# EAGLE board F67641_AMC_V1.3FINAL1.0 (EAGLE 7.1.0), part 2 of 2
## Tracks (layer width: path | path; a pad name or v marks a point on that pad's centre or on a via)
+5..12V
  Top 0.406: C55.1 133.85,154.74 U3.3 | U3.1 135.28,152.84 135.74,153.3 135.74,154.64 C55.1 | C54.1 137.64,157.46 arc45 137.56,157.28 D6.1 D7.1 135.79,154.67 arc-45 C55.1
ACT  (via drill 0.4)
  Top 0.254: 117.74,138.48 112.19,144.18 | 112.19,144.18 107.6,148.88 107.6,166.33 100.71,173.22 100.71,173.27 59,173.27 LED_ACT.K 54.01,171.54 53.5,172.05 53.5,174.21 54.38,175.1 v58.3,175.1 | 112.19,144.18 117.86,138.51 117.86,104.64 109.86,96.64 U4.51
  Top 0.61: U5.2 39.27,177.2 42.82,180.75 65.4,180.8 ACT.2
  Bottom 0.254: v58.3,175.1 61.57,178.37 62.97,178.37 ACT.2
AGND_I1  (via drill 0.4)
  Top 0.813: U$13.2 140.64,29.69 C35.2 | U$16.7 140.57,44.4 C39.2 138.57,44.36 U$16.6 140.48,50.23 140.75,50.5
  other vias: 121.67,20.51 124.21,20.51 126.75,20.51 130.56,20.56 135.64,21.83 135.64,19.8 140.47,21.83 140.47,20.05 133.86,28.69 133.86,26.91 143.51,28.69 143.51,26.66 122.69,22.59 122.43,27.42 121.67,31.99 123.45,31.99 117.61,33.52 117.61,36.82 117.61,41.14 117.61,44.69 117.61,47.99 117.61,50.28 119.38,47.99 119.38,45.45 123.45,38.09 122.18,38.09 122.18,36.82 123.45,36.82 120.65,41.9 122.43,41.9 124.46,41.9 126.75,34.28 128.81,34.28 134.62,40.37 134.37,30.98 141.48,31.48 143.51,31.48 143.51,33.52 143.51,37.83 140.97,37.83 140.97,39.87 143.51,39.87 129.62,51.42 130.84,51.42 132.06,51.42 133.28,51.42 129.62,50.46 130.84,50.46 132.06,50.46 133.28,50.46 129.87,43.04 134.5,50.31 128.78,38.09 130.18,38.14 131.55,38.11 133.68,38.06 128.81,35.73 130.23,35.73 131.5,35.73 133.71,35.73
  pour Bottom: 115.9,52.16 144.53,52.16 144.53,17.89 115.9,17.89
  pour Top: 115.9,52.16 144.53,52.16 144.53,17.89 115.9,17.89
AGND_I2  (via drill 0.4)
  Top 0.813: U$7.2 90.64,29.69 C44.2 | U$8.7 90.57,44.4 C45.2 88.57,44.36 U$8.6 90.73,50.23 90.76,50.25
  other vias: 70.87,20.51 74.43,20.51 72.65,22.59 76.97,20.51 81.03,20.51 84.33,31.23 91.19,31.48 93.48,31.48 93.48,34.02 93.48,37.07 91.19,37.07 91.19,39.87 93.48,39.87 83.87,40.12 84.84,49.26 72.39,28.44 71.89,31.99 73.41,31.99 72.14,36.82 73.16,36.82 72.14,39.1 73.16,39.1 70.87,41.9 72.65,41.9 74.43,41.9 76.71,34.53 79.25,34.53 67.06,37.33 67.06,41.39 67.06,44.18 69.35,45.45 69.35,47.74 67.06,47.74 67.06,49.77 85.09,20.31 90.68,20.05 85.09,22.09 90.68,22.09 84.2,26.4 84.18,28.69 93.48,26.15 93.48,28.69 79.53,51.42 80.75,51.42 81.97,51.42 83.19,51.42 79.53,50.46 80.75,50.46 81.97,50.46 83.19,50.46 79.96,43.09 79.2,37.81 80.6,37.81 81.72,37.78 79.23,35.93 80.6,35.9 81.74,35.9 83.87,38.04 83.93,35.7
  pour Bottom: 65.9,52.16 94.53,52.16 94.53,17.89 65.9,17.89
  pour Top: 65.9,52.16 94.53,52.16 94.53,17.89 65.9,17.89
AGND_I3  (via drill 0.4)
  Top 0.813: U$15.6 38.48,50.15 38.48,44.45 C50.2 40.57,44.4 U$15.7 | 40.82,50.18 40.7,50.3 | U$14.2 40.64,30.93 40.06,31.51 C48.2
  other vias: 22.81,42.05 24.67,42.05 20.6,42.05 21.85,39.79 21.87,36.95 42.73,39.18 42.65,36.01 40.49,36.01 40.54,39.18 17.4,44.56 17.4,47.28 17.4,49.52 17.4,33.16 27.49,33.64 28.96,39.1 17.4,36.67 17.4,41.24 30.79,39.1 29.77,33.64 34.93,49.31 30.51,20.51 26.88,20.51 23.91,20.51 21.01,20.51 18.83,20.51 19.79,47.41 19.79,45.15 30.33,42.69 33.74,31.1 34.22,41.44 24.29,49.31 23.37,39.79 23.37,36.95 21.87,32.12 23.42,32.14 22.66,29.1 22.64,22.49 42.65,33.19 40.62,33.19 42.65,31.84 34.9,22.19 40.75,22.19 40.75,19.9 34.9,19.9 42.65,27.27 42.65,28.99 33.74,26.51 33.74,29.05 29.42,51.42 30.64,51.4 29.42,50.46 30.64,50.46 31.86,51.4 31.86,50.46 33.07,51.4 33.07,50.46 28.91,35.5 30.1,35.5 31.17,35.52 28.91,37.88 30.15,37.86 31.2,37.86 33.1,37.86 33.1,35.85
  pour Bottom: 15.9,52.16 44.53,52.16 44.53,17.89 15.9,17.89
  pour Top: 15.9,52.16 44.53,52.16 44.53,17.89 15.9,17.89
AMC_CLKIN  (via drill 0.4)
  Top 0.254: 123.36,67.64 123.37,67.65 | U4.47 99.15,92.43 96.83,90.11 96.83,89.55
  Top 0.61: U$3.CLKIN 73.41,61.06 73.41,65.19 74.3,66.08 74.3,68.14 JP2.2 68.06,68.19 R16.2 | JP3.2 23.37,67.17 U$4.CLKIN | JP1.2 123.37,67.65 U$2.CLKIN | v94.87,77.9 96.83,79.86 96.83,89.55
  Bottom 1.016: 75.85,77.9 v94.87,77.9 122.05,77.9 124.67,75.28 JP1.2 | JP3.2 25,75.15 27.77,77.9 72.46,77.9 73.55,76.81 | JP2.2 74.25,76.11 | 74.25,76.11 74.25,76.3 75.85,77.9 | 73.55,76.81 74.25,76.11 | 69.52,77.9 74.64,77.9 | 75.85,77.9 74.64,77.9 | 74.64,77.9 73.55,76.81
AUXVCC1
  Top 0.254: C4.1 79.44,101.31 C5.1 82.99,101.31 R6.2 83.05,101.26 84.15,101.26 85.77,99.64 U4.19
AUXVCC2
  Top 0.254: 74.72,101.11 C7.1 | 74.74,101.13 C7.1 | C7.1 C6.1 77.86,101.34 R5.2 | U4.18 85.95,100.15 83.95,102.15 78.08,102.15 77.91,101.97 R5.2 | 77.91,101.35 R5.2
AUXVCC3
  Top 0.254: 91.28,92.22 C58.1 | 91.33,90.44 C59.1 | U4.26 88.66,93.83 89.13,93.36 90.14,93.36 C58.1 | C59.1 C58.1 | R7.2 91.25,90.33 C59.1
AVCC  (via drill 0.2, 0.6)
  Top 0.254: U4.9 83.84,104.64 81.79,106.69 C29.1
  Top 0.406: v44.67,108.35 D46.C | v44.67,98.85 D48.C | v44.67,117.85 D44.C
  Top 0.61: v44.67,108.35 R123.1 | v44.67,117.85 R117.1 | v44.67,98.85 R127.1
  Top 0.813: 44.67,97.35 v44.67,98.85 | C29.1 C31.1 75.12,108.33 56.3,127.16 R36.2 44.67,127.15 v44.67,125.85
  Bottom 0.813: v44.67,98.85 v44.67,108.35 v44.67,117.85 v44.67,125.85
AVDD_I1
  Top 0.61: D3.C 117.25,27.56 117.25,20.28 118.67,18.86 131.73,18.86 132.52,19.67 132.52,27.17 | U$2.AVDD 127.18,49.82 127.75,49.25 129.19,49.25 C12.1 CSEL1.1 130.97,47.28 132.52,45.75 132.52,28.16 | D4.C 131.9,27.64 131.91,27.65 132.01,27.65 | 132.01,27.65 132.52,28.16 | 132.52,27.17 132.01,27.65 | 132.52,28.16 132.52,27.17
AVDD_I2
  Top 0.61: 82.66,28.13 82.66,45.63 81,47.28 CSEL2.1 C19.1 79.25,49.19 77.96,49.19 77.18,49.96 U$3.AVDD | D1.C 67.06,27.37 67.06,20.16 68.25,18.96 81.84,18.96 82.66,19.77 82.66,26.99 82.13,27.51 82.13,27.61 | D5.C 78.08,27.61 82.13,27.61 | 82.13,27.61 82.66,28.13 | 82.66,27.09 82.66,28.13
AVDD_I3
  Top 0.61: D13.C 17.28,19.7 18.09,18.89 31.17,18.89 31.74,19.46 32.08,19.8 32.19,19.9 32.19,27.15 31.7,27.64 | U$4.AVDD 27.18,49.77 27.77,49.19 29.25,49.19 C21.1 CSEL3.1 30.79,47.28 32.19,45.89 32.19,28.13 | D15.C 31.7,27.64 | 31.7,27.64 32.19,28.13 | 32.19,28.13 32.19,27.06
BTN1
  Top 0.254: U4.46 98.64,95.96 98.86,96.18 103.41,96.18 105.72,93.86 R49.2
  Top 0.61: BTN1.2 122.1,93.85 118.93,93.85 R49.2
COM0  (via drill 0.2)
  Top 0.254: U4.32 91.66,96.91 94.75,100 94.75,107.25 v95.5,108
  Bottom 0.254: LCD1.COM0 94.49,161.57 106.25,161.57 112.75,155.07 112.75,111.5 108.5,107.25 98.5,107.25 97.5,108.25 95.75,108.25 v95.5,108
COM1  (via drill 0.2)
  Top 0.254: U4.33 92.17,96.67 95.25,99.75 95.25,106.5 96.25,107.5 v97.25,107.5
  Bottom 0.254: LCD1.COM1 96.53,162.07 106.5,162.07 113.25,155.32 113.25,111.25 108.75,106.75 98,106.75 v97.25,107.5
COM2  (via drill 0.2)
  Top 0.254: U4.34 92.65,96.4 96,99.75 96,106 v96.25,106.25
  Bottom 0.254: LCD1.COM2 98.57,162.57 106.75,162.57 113.75,155.57 113.75,111 109,106.25 v96.25,106.25
COM3  (via drill 0.2)
  Top 0.254: v97.25,105 96.75,105 96.5,104.75 96.5,99.5 93.16,96.16 U4.35
  Bottom 0.254: LCD1.COM3 100.61,163.07 105.25,163.07 106.98,163.09 114.25,155.82 114.25,110.75 109.2,105.7 97.97,105.7 97.27,105 v97.25,105
CUR1+
  Top 0.61: I1+.TP 120.68,23.23 D3.A D11.C 120.68,33.75 TVS2.C R/L9.2
CUR1+1
  Top 0.61: I2+.TP 70.68,23.23 D1.A D2.C 70.68,33.75 TVS1.C R/L1.2
CUR1+2
  Top 0.61: R/L3.2 TVS3.C 20.68,33.75 D14.C D13.A 20.68,23.23 I3+.TP
CUR1-
  Top 0.61: I1-.TP 124.65,23.14 D4.A 124.65,29.81 D12.C 124.62,33.87 TVS2.A R/L10.2
CUR1-1
  Top 0.61: I2-.TP 74.65,23.14 D5.A 74.62,27.67 D10.C 74.64,29.86 TVS1.A R/L2.2
CUR1-2
  Top 0.61: I3-.TP 24.65,23.14 D15.A 24.62,27.67 D35.C 24.62,33.87 TVS3.A R/L4.2
DRESET  (via drill 0.2)
  Top 0.254: U4.100 88.66,104.55 v91.88,101.33
  Bottom 0.254: v91.88,101.33 94.64,98.56 126.16,98.56 arc-45 126.34,98.49 128.43,96.41 128.43,89.65 131.07,87.01 131.5,87.01 137.42,87.01 JP5.2
DTCK  (via drill 0.2)
  Top 0.254: U4.99 89.14,105.06 v91.37,102.83
  Bottom 0.254: JP6.2 137.44,89.67 129.7,89.67 129.11,90.26 129.11,97.07 127.05,99.13 arc45 126.87,99.2 95.03,99.2 94.85,99.38 94.85,99.4 91.42,102.83 v91.37,102.83
DTDI  (via drill 0.2)
  Top 0.254: U4.97 90.16,106.48 v93.22,103.42
  Bottom 0.254: JP8.2 137.39,94.96 133.63,94.96 132.03,94.96 130.84,96.15 130.84,98.95 129.52,100.27 arc45 129.34,100.34 96.3,100.34 v93.22,103.42
DTDO  (via drill 0.2)
  Top 0.254: U4.96 90.67,107.22 v93.3,104.53
  Bottom 0.254: JP9.2 137.47,97.68 133.21,97.68 arc-45 133.03,97.75 126.47,104.31 115.58,104.31 arc45 115.4,104.23 112.12,100.95 96.85,100.95 95.46,102.35 95.46,102.38 v93.3,104.53
DTMS  (via drill 0.2)
  Top 0.254: U4.98 89.65,105.92 v91.5,104.08
  Bottom 0.254: JP7.2 137.6,92.5 133.35,92.5 130.71,92.5 129.95,93.26 129.95,97.85 128.15,99.66 arc45 127.97,99.73 95.79,99.73 95.18,100.34 95.18,100.37 91.5,104.05 v91.5,104.08
DVCC  (via drill 0.2, 0.4, 0.6)
  Top 0.254: U4.21 84.82,98.65 84.43,98.26 84.43,95.72 82.83,94.12 78.29,94.12 77.96,94.45 C17.1
  Top 0.406: v60.27,166.27 R58.1 | v70.27,166.27 R22.1 | v80.27,166.27 R57.1 | v90.27,166.27 R21.1 | v100.27,166.27 R20.1 | 90.53,61.07 U$8.2 | U$2.DVDD 122.1,61.9 | 122,63.48 C24.1 | 140.57,63.17 C51.1 140.5,63.24 | 80.32,177.23 80.35,177.26 80.81,177.26 arc-45 80.88,177.23 | 128.86,109.4 arc-45 128.79,109.43 128.39,109.83 | 128.86,109.53 128.86,110.32 arc45 128.78,110.5 | 128.25,109.97 128.25,110.3 arc-45 128.32,110.48 128.86,111.01 | 121.64,128.08 v121.62,128.11 121.71,128.02 C65.2 138.38,128.09 U1.1
  Top 0.61: 90.53,61.07 C46.1 90.53,64.61 90.03,65.1 U$6.2 90.03,66.98 89.72,67.3 84.63,67.3 C47.1 84.43,67.19 84.43,69.51 v84.46,69.53 | U$8.2 U$8.3 | 71.86,63.23 C26.1 | v120.73,68.31 122.09,66.96 C23.1 C24.1 122.1,63.55 122.1,61.9 | v107.06,80.58 v107.06,73.88 107.19,74 132.34,74 134.48,71.86 C42.1 139.68,67.2 139.75,67.27 140.03,66.99 U$10.2 140.03,65.29 140.49,64.83 140.49,63.24 C51.1 | 71.83,66.74 v71.91,66.81 | 68.51,80.28 68.79,80.56 | 71.85,66.75 v71.91,66.81 | C22.1 59.41,66.86 CLOCK_GENERATOR.4 59.43,68.53 v59.34,68.62 | U$15.3 U$15.2 40.57,63.17 C41.1 | 40.5,63.24 C41.1 | U$16.3 U$16.2 140.5,61.1 140.5,63.24 | C41.1 40.52,63.22 40.52,64.53 40.03,65.01 U$12.2 40.03,67.02 39.68,67.37 36.63,67.37 35.11,65.85 33.82,65.85 C52.1 33.73,65.94 v33.73,68.01 | U$4.DVDD C34.1 C27.1 22.11,70.51 23.93,72.33 33.71,72.33 v33.79,72.4 33.79,77.69 | 60.63,80.56 59.36,79.29 59.36,79.39 58.17,80.58 | v71.91,74.51 71.91,78.98 | 71.91,78.98 71.99,79.06 72.14,79.06 | 71.91,78.98 71.86,78.98 70.23,80.56 | 72.14,79.06 73.64,80.58 | 72.14,79.36 71.4,80.1 71.35,80.1 | 72.14,79.36 72.14,79.8 72.9,80.56 | 72.14,79.06 72.14,79.36 | v59.39,74.72 59.39,80.45 60,80.56 60.23,80.56 | v84.46,76.29 84.46,80.56 v84.43,80.58 | v71.91,66.81 72.04,66.69 C25.1 72.06,64.94 C26.1 | U$3.DVDD 72.1,63.22 C26.1 | U5.1 38.7,175.93 C66.1 40.56,176 41.53,175.02 41.53,173.34 42.27,172.61 43.82,172.61 43.84,172.63 | 44.66,171.87 44.66,173.16 44.52,173.31
  Top 0.813: DVCC.1 DVCC.2 DVCC.3 DVCC.4
  Top 1.27: 78.57,177.23 52.35,177.26 48.01,177.26 44.66,174.47 44.66,173.45 44.52,173.31 43.84,172.63 44.66,171.82 v44.66,166.05 R36.1 | 78.57,177.23 80.32,177.23 | 61.93,82.69 61.93,90.49 66.65,95.21 C16.1 C17.1 | 61.93,82.69 61.93,82.51 60.23,80.56 60.63,80.56 62.82,80.56 | 33.79,77.69 36.66,80.56 60,80.56 | 70.23,80.56 68.79,80.56 66.6,80.56 | v84.43,80.58 73.64,80.58 73.56,80.56 | 73.46,80.56 72.9,80.56 69.68,80.56 | DVCC.1 80.35,179.06 | 80.35,179.06 82.17,177.23 | 80.35,179.06 80.35,179.01 78.57,177.23 | 79.81,178.04 80.55,178.04 80.57,178.02 80.37,177.81 80.37,177.23 80.88,177.23 82.17,177.23 | R51.1 arc45 131.5,95.84 131.5,98.56 128.93,101.13 arc-45 128.86,101.31 128.86,109.4 | 127.62,110.6 127.5,110.48 arc-45 127.32,110.4 121.52,110.4 118.91,107.8 v118.91,97 R49.1 118.85,95.5 | 127.62,110.6 128.86,111.86 128.86,113.55 130.61,115.28 JP10.2 arc45 133.69,115.25 135.39,115.25 | 128.7,109.52 128.39,109.83 128.25,109.97 127.62,110.6 | 128.86,112.18 128.86,111.01 128.86,109.53 arc-45 128.66,109.61 | 82.17,177.23 102.39,177.28 109.53,177.28 v117.3,169.51 | 44.66,173.72 44.66,171.87 | 61.93,82.69 66.6,80.56 | 66.6,80.56 62.82,80.56 | 62.82,80.56 61.67,81.7
  Bottom 0.406: v121.62,128.11 118.01,128.11 117.2,128.92
  Bottom 0.61: v33.73,68.01 33.73,72.35 v33.79,72.4 | v71.91,66.81 v71.91,74.51 | v84.46,69.53 v84.46,76.29 | v59.34,68.62 59.34,74.66 v59.39,74.72 | v107.06,73.88 107.06,70.4 109.15,68.31 v120.73,68.31 | v44.66,166.05 44.88,166.27 v60.27,166.27 v70.27,166.27 v80.27,166.27 v90.27,166.27 v100.27,166.27
  Bottom 1.27: v84.43,80.58 v107.06,80.58 111.75,80.58 113.75,82.58 113.75,95.25 115.5,97 v118.91,97 | JP10.2 119.79,115.28 117.2,117.87 117.2,126.89 | 117.2,126.89 118.32,128 | v117.3,169.51 117.3,129.49 | 117.3,129.49 118.32,128 | 117.3,129.49 117.2,128.92 117.2,126.89 | 118.32,128 117.83,128 117.4,128.44
EXT
  Top 1.27: JTAG.4 152.23,101.87 153.44,103.09 153.44,107.25 148.95,111.75 142.14,111.75 136.15,117.74 arc45 135.97,117.82 JP10.3
EXT1
  Top 0.813: U$13.1 135.56,30.15 C35.1 136.93,35.06 AMC1PWR.1
EXT2
  Top 0.813: U$7.1 85.56,30.15 C44.1 86.92,35.06 AMC2PWR.1
EXT3
  Top 0.305: 37.04,31.62 C48.1
  Top 0.813: U$14.1 35.56,30.15 C48.1 | 37.04,31.62 AMC3PWR.1
GND  (via drill 0.3, 0.4)
  Top 0.254: 86.39,105.12 U4.8 84.5,105.12 83.77,105.86 83.77,106.9 v83.52,107.15 | U4.22 88.52,98.14 v88.87,97.79 | C65.1 138.36,124.04 138.33,124.02
  Top 0.406: U1.4 142.19,124.4
  Top 1.016: L6.2 30.6,82.1 37.25,88.75
  other vias: 71.75,150.07 59.25,150.07 84.25,143.07 71.75,143.07 59.25,143.07 80.76,120.63 50.34,91.5 38.51,82.23 38.51,84.23 38.51,86.72 40.46,82.23 40.46,84.23 40.46,86.72 42.26,82.23 42.26,84.23 42.26,86.72 103.96,183.59 76.93,182.67 42.09,126.12 42.09,124.87 42.1,123.8 41.92,110.28 24.52,63 20.27,66.75 20.27,68 27.02,63 27.02,65 29.02,63 29.02,65 29.64,61.27 31.52,61.25 42.77,65.43 33.02,62.25 46.01,65.43 37.77,66.25 36.14,69 42.77,68.5 37.02,63.25 66.49,63.09 66.49,65.2 78.52,63 78.27,64.5 79.52,61.75 79.77,63.75 86.52,63.25 75.02,64 80.77,61 82.02,61 86.52,69.75 86.77,66 95.66,69.67 95.66,66.75 116.49,66.75 116.49,63.29 124.77,64.25 128.27,65 129.77,65 128.27,63.75 129.77,63.75 130.27,61.5 132.02,61.5 133.27,61.5 137.07,69 137.07,66.27 144.77,69 144.77,66.25 147.56,66.25 137.07,63.25 37.4,156.73 37.4,151.6 37.4,132.62 39.09,119.17 42.09,119.12 39.09,116.12 42.09,116.12 38.59,110.37 85.28,120.58 80.76,117.08 85.28,117.08 20.27,72.82 22.55,72.82 20.24,77.09 22.55,77.09 29.44,74.37 31.52,74.37 31.52,76.4 29.44,76.4 36.14,71.93 36.14,76.45 36.14,74.14 57.48,76.45 57.48,71.93 57.48,74.14 61.85,76.45 69.77,76.45 61.85,74.14 61.85,71.93 69.77,74.14 69.77,71.93 49.22,65.43 52.5,65.43 56.26,63.09 60.91,63.09 64.26,63.09 64.26,65.2 66.01,83.24 69.36,83.24 58.29,83.16 83.77,84.56 87.58,84.53 87.63,82.63 83.74,82.65 81.73,75.97 81.73,73.02 78.81,69.34 81.73,69.34 100.07,82.37 100.07,85.95 100.07,89.89 97.63,92.43 102.05,82.37 102.05,85.95 102.05,89.89 101.83,93.9 91.14,73.02 95.66,73.02 95.66,75.97 91.14,75.97 102.24,75.97 104.99,75.97 102.24,73.81 104.91,73.81 101.99,66.75 101.99,63.29 95.66,63.29 101.99,69.67 110.04,63.29 110.04,66.75 109.73,75.97 120.58,75.97 120.58,79.17 113.77,79.22 109.94,73.07 120.68,73.04 110.04,69.67 120.73,69.67 129.17,72.54 130.61,72.54 130.61,70.28 132.11,70.17 137.07,73.4 137.07,70.81 38.51,88.95 40.46,88.95 42.26,88.95 38.51,90.98 40.46,90.98 42.26,90.98 147.56,69 98.76,74.27 100.06,79.12 97.7,79.12 102.06,79.17 104.96,79.12 95.93,93.19 97.63,93.45 101.88,92.84 101.62,94.92 91.01,97.84 90.78,100.43 93.19,108.79 102.97,112.6 101.85,112.6 50.34,83.16 38.67,103.69 42.04,104.2 97.89,89.89 97.89,86.03 97.89,82.37 102.92,91.74 104.29,85.95 104.29,82.42 95.27,82.35 95.27,85.93 95.27,89.81 67.79,100.28 69.31,100.25 88.19,92.71 102.97,111.12 101.85,111.15 145.41,124.18 148.46,124.18 137.71,124.49 136.77,124.49 143.58,124.18 103.96,181.43 76.93,184.19 37.4,183.2 123.82,124.49 37.4,181.2 37.4,172.66 31.34,71.42 79.5,98.32 81.28,98.32 77.82,98.37 37.4,170.5 146.81,124.18 84.07,149.85 127.33,84.73 127.38,87.34 127.12,107.69 39.33,172.66 39.33,170.3 39.33,183.18 39.33,181.2 103.96,185.08 76.96,181.33 127.12,124.49 130.3,124.49 134.06,124.49 136.75,123.29 137.71,123.29 143.58,123.29 145.38,123.29 146.78,123.29 148.48,123.27 59.21,117.71 59.24,116.32 53.52,122.11 55.25,122.11 53.62,125.51 55.35,125.49 55.58,116.14 53.65,116.11 53.75,112.05 55.55,112.02 53.7,106.82 55.55,106.82 59.49,108.06 59.49,106.69 53.75,102.5 55.6,102.5 53.78,97.42 55.6,97.39 59.52,98.84 59.49,97.6 103.96,175.31 51.07,175.15
  pour Bottom (isolate 0.1): 36.61,186.65 133.45,186.65 arc45 133.63,186.68 133.63,172.39 arc-45 133.58,172.33 119.27,172.33 119.27,124.93 155.17,124.93 155.17,60.52 arc-45 155.17,60.49 18.6,60.49 18.6,80.76 36.61,80.76
  pour Top (isolate 0.1): 36.61,186.65 133.45,186.65 arc-45 133.63,186.65 133.63,186.68 133.63,172.39 arc-45 133.56,172.3 133.58,172.33 119.27,172.33 119.27,124.93 155.17,124.93 155.17,60.49 18.6,60.49 18.6,80.76 36.61,80.76
GND_RS232  (via drill 0.4)
  Top 0.406: v130.97,140.83 129.87,140.83 129.29,141.42 129.29,142.22 C63.1
  other vias: 128.66,154.98 140.77,160.34 140.75,158.46 140.77,162.14 140.77,152.01 138.92,152.01 132.31,158.84 132.31,157.01 128.66,136.44 133.46,136.44 145.04,136.44 148.64,136.44 147.1,145.4 150.27,145.4 144,164.45 153.42,164.45 133.46,140.88 138.87,140.32 152.76,136.44
  pour Bottom: 155.32,169.05 141.76,169.05 141.76,163.45 arc-45 141.74,163.39 141.74,163.16 127.75,163.16 127.75,135.62 arc-45 127.75,135.5 155.32,135.5
  pour Top: 155.32,169.05 141.76,169.05 141.76,163.45 arc-45 141.74,163.39 141.74,163.16 127.75,163.16 127.75,135.62 arc-45 127.75,135.5 155.32,135.5
INT
  Top 1.27: 148.72,107.66 148.54,107.84 | JTAG.2 150.91,105.47 148.9,107.48 148.72,107.66 | JP10.1 JP10.1 arc45 133.56,112.56 133.56,109.74 135.49,107.81 arc45 135.67,107.73 148.54,107.73 arc-45 148.72,107.66
LDO_IN1  (via drill 0.4)
  Top 0.305: 136.91,37 AMC1PWR.2
  Top 0.61: U$2.LDO_IN 125.91,47.31 CSEL1.3 125.94,44.49 127.49,42.94 127.49,37.58 128.2,36.87 v129.7,36.87 | AMC1PWR.2 v134.37,36.87
  Bottom 0.61: v134.37,36.87 v129.7,36.87
LDO_IN2  (via drill 0.4)
  Top 0.305: 87.01,36.89 AMC2PWR.2
  Top 0.61: U$3.LDO_IN 75.91,47.31 CSEL2.3 75.94,44.3 77.4,42.84 77.4,37.53 v78.06,36.87 | v83.95,36.87 AMC2PWR.2
  Bottom 0.61: v78.06,36.87 v83.95,36.87
LDO_IN3  (via drill 0.4)
  Top 0.61: U$4.LDO_IN 25.91,47.31 CSEL3.3 25.94,44.36 27.41,42.89 27.41,37.58 v27.97,37.02 | AMC3PWR.2 v33.73,36.87
  Bottom 0.61: v33.73,36.87 28.12,36.87 v27.97,37.02
LED_PHASE_1  (via drill 0.2)
  Top 0.254: U4.40 95.65,97.65 96.5,98.5 97,98.5 97.5,99 97.5,103.5 v97.5,103.78
  Bottom 0.254: LED_PHASE_1.K 67.29,171.54 69.52,173.77 99.91,173.77 | v97.5,103.78 109.5,103.75 115.75,110 115.75,169.38 111.36,173.77 99.91,173.77 | 99.91,173.77 99.9,173.78
LED_PHASE_2  (via drill 0.2)
  Top 0.254: U4.41 96.15,97.4 96.5,97.75 98.5,97.75 99,98.25 v99,104.5
  Bottom 0.254: LED_PHASE_2.K 77.29,171.54 79.02,173.27 110.85,173.27 111.13,172.99 111.53,172.58 115.25,168.87 115.25,110.25 109.5,104.5 v99,104.5
LED_PHASE_3  (via drill 0.2)
  Top 0.254: U4.42 96.66,96.41 97.25,97 99,97 100.5,98.5 v100.5,105.1
  Bottom 0.254: LED_PHASE_3.K 87.29,171.54 88.52,172.77 110.31,172.77 110.39,172.68 110.82,172.25 114.75,168.32 114.75,110.5 109.33,105.08 100.53,105.08 v100.5,105.1
LINE_1
  Top 0.813: L1.1 20.94,157.84 19.5,157.84 R1.2 14.93,157.84 LINE_1.TP
  Top 1.016: 18.74,157.76 R1.2 | 19.34,158 19.5,157.84
LINE_2
  Top 1.016: LINE_2.TP 18.8,129.86 R2.2 20.94,129.84 L3.1
LINE_3
  Top 0.813: L5.1 21.86,100.62 R3.2 16.2,100.62 LINE_3.TP
  Top 1.016: 2.75,113.66 LINE_3.TP
LINE_V1
  Top 0.406: D45.C 44.67,121.83 44.75,121.75 44.67,121.67 D44.A
  Top 0.813: R119.2 R118.2 | R119.2 46.82,123.25 | 46.82,123.25 R116.1 | R101.1 35.93,156.11 39.81,152.24 39.81,123.19 41.25,121.75 44.75,121.75 46.72,121.75 R119.2 | 46.82,123.25
LINE_V2
  Top 0.406: D46.A 44.67,112.35 D47.C
  Top 0.813: 45.37,112.35 44.67,112.35 39.51,112.35 36.88,114.97 36.88,126.63 35.49,128.03 33.25,128.03 R108.1 | 45.37,112.35 R122.2 | R122.2 R121.2 | R122.2 R120.1 | 45.32,112.31 45.37,112.35
LINE_V3
  Top 0.406: D49.C 44.67,102.85 D48.A
  Top 0.813: 43.67,102.85 44.67,102.85 44.76,102.85 | 44.76,102.85 44.81,102.85 | 44.81,102.85 R126.2 | R126.2 R125.2 | R126.2 R124.1 | 44.74,102.83 44.76,102.85 | 36.48,98.92 35.62,98.92 35.44,99.1 | R115.1 36.45,98.89 36.48,98.92 | 36.48,98.92 37.88,98.92 41.79,102.83 44.79,102.83 44.81,102.85
MSP_SD_DIN_I1
  Top 0.254: 125.94,61.05 U$2.DOUT | U4.50 100.64,95 100.64,92.55 103.13,90.06 103.13,89.14 103.1,89.12
  Top 0.61: 125.94,61.05 125.94,63.21 127.21,64.48 JP1.1 | 103.46,72.45 103.13,72.78 103.1,72.81 103.1,89.12
  Top 0.813: JP1.1 127.21,70.62 126.19,71.64 105.52,71.64 104.27,71.64 103.46,72.45
MSP_SD_DIN_I2
  Top 0.254: 76.86,68.11 JP2.1 | 100.17,73.79 99.69,73.31 | U4.49 100.17,92.08 100.99,91.25 100.99,90.82
  Top 0.61: 76.86,68.11 76.86,63.39 75.91,62.43 U$3.DOUT | 100.99,90.82 100.99,74.61
  Top 0.813: JP2.1 76.79,70.55 77.86,71.62 98,71.62 99.69,73.31 100.99,74.61
MSP_SD_DIN_I3
  Top 0.254: U4.48 99.66,91.72 99.11,91.17 99.11,90.62
  Top 0.61: U$4.DOUT 25.91,67.17 JP3.1 | 99.11,90.62 99.11,76.44
  Top 0.813: 99.11,76.44 96.98,74.31 75.06,74.31 71.07,70.32 28.86,70.32 JP3.1
N$1
  Top 0.61: CSEL1.2 127.64,44.99 C11.1
N$2
  Top 0.813: AMC1PWR.3 137.04,39.46 136.5,40 136.5,41.45 U$1.C C39.1 142.53,41.48 U$19.C
N$3  (via drill 0.4)
  Top 0.61: ISO_PULSE.1 18.5,175.93 23.73,175.93 v23.75,175.96 | v23.52,180.86 23.52,182.13 24.59,183.2 28.3,183.2 29.01,182.49 29.01,181.58 C67.1 | U5.8 24.26,175.93 | 24.26,175.93 23.78,175.93 v23.75,175.96 | v23.75,175.96 24.24,175.96 24.26,175.93
  Bottom 0.61: v23.52,180.86 23.52,176.19 v23.75,175.96
N$4
  Top 0.254: U4.29 90.16,94.03 90.5,93.69 92.31,93.69 92.75,93.25 C49.1
N$5
  Top 0.254: R20.2 96.67,168.15 LED_REACT.A
N$6
  Top 0.254: R21.2 86.42,168.15 LED_PHASE_3.A
N$7
  Top 0.254: R22.2 66.42,168.15 LED_PHASE_1.A
N$8
  Top 0.61: R/L9.1 R135.2
N$9
  Top 0.406: U2.4 131.24,144.59 arc-45 C57.1
N$11
  Top 0.61: U5.7 17.23,177.2 ISO_PULSE.2
N$12
  Top 0.61: U5.6 15.95,178.47 ISO_PULSE.3
N$13
  Top 0.61: R/L10.1 124.64,40.16 R136.2
N$14
  Top 0.61: R135.1 118.75,40.26 118.75,42.75 119.6,43.6 C2.1 121.75,43.64 121.75,47.25 120.83,48.17 U$2.AINP
N$15
  Top 0.61: R136.1 126.25,40.28 126.25,42.75 125.4,43.6 C2.2 123.41,47.09 122.1,48.4 U$2.AINN
N$16
  Top 0.61: R/L1.1 R137.2
N$17
  Top 0.813: AMC2PWR.3 87.04,39.45 86.42,40.07 86.42,41.41 U$5.C C45.1 92.53,41.48 U$9.C
N$18
  Top 0.61: CSEL2.2 77.64,44.99 C13.1
N$19
  Top 0.61: R/L2.1 74.64,40.16 R138.2
N$20
  Top 0.61: 71.68,43.57 C3.1 | R137.1 68.84,42.74 69.6,43.5 71.61,43.5 C3.1 | C3.1 71.68,43.62 71.68,47.77 70.83,48.62 U$3.AINP
N$21
  Top 0.61: R138.1 76.31,40.22 76.31,42.71 75.42,43.6 C3.2 73.44,43.63 73.44,47.38 72.1,48.72 U$3.AINN
N$22
  Top 0.406: C57.2 arc45 129.26,144.58 129.26,143.85 129.55,143.57 arc45 129.72,143.5 131.45,143.5 131.81,143.86 arc-45 131.99,143.93 U2.5
N$23
  Top 0.61: R/L3.1 R139.2
N$24
  Top 0.406: C60.1 134.69,146.74 134.5,146.55 U2.1
N$25
  Top 0.61: R/L4.1 24.64,40.16 R140.2
N$26
  Top 0.406: C60.2 136.39,146.36 135.28,145.25 133.07,145.25 U2.3
N$27
  Top 0.61: U$4.AINP 20.81,51.63 20.81,49.06 21.71,48.16 C10.1 19.77,43.6 18.84,42.67 R139.1
N$28
  Top 0.406: U2.12 137.75,143.93 arc45 137.57,143.86 137.11,143.4 137.11,140.12 arc45 137.19,139.94 139.34,137.8 139.53,137.6 | 139.6,137.42 arc45 139.53,137.6 | U1.7 139.65,137.48 139.53,137.6
N$29
  Top 0.61: U$4.AINN 22.13,51.63 22.13,49.16 23.41,47.88 C10.2 23.43,43.57 25.48,43.57 26.36,42.7 R140.1
N$30
  Top 0.61: C20.1 27.68,47.24 CSEL3.2
N$31
  Top 0.61: R16.1 61.56,66.81 CLOCK_GENERATOR.3
N$32
  Top 0.813: U$16.5 136.57,45.36 U$1.A
N$33
  Top 0.406: U2.11 140.28,143.3 arc-45 140.46,143.22 140.58,143.1 140.8,142.89 | 140.87,142.71 arc45 140.8,142.89 | U1.6 140.92,142.76 140.8,142.89
N$34
  Top 0.406: 133.63,100.09 133.63,101.36 135.21,102.93 140.09,102.93 JP4.1
  Top 0.61: R48.2 133.63,100.09
N$35
  Top 0.813: U$16.8 142.57,45.48 U$19.A
N$36
  Top 0.406: U2.2 C62.2
N$37
  Top 0.813: U$5.A 86.48,50.14 U$8.5
N$38
  Top 0.61: U$16.4 135.41,61.03 134.68,61.76 134.68,64.38 135.54,65.24 138.66,65.24 139.08,65.66 U$10.1
N$39
  Top 0.61: U$10.3 140.98,65.64 142.5,64.12 142.5,61.1 U$16.1
N$40
  Top 0.406: C63.2 131.97,143.22 arc-45 132.15,143.3 U2.6
N$42
  Top 0.813: U$9.A 92.65,50.15 U$8.8
N$43
  Top 0.61: U5.5 29.05,179.74 C67.2 15.21,179.83 ISO_PULSE.4
N$44
  Top 0.254: R58.2 56.42,168.15 LED_ACT.A
N$45
  Top 0.406: 86.62,61.08 U$8.4
  Top 0.61: U$6.1 89.08,65.5 88.04,64.45 85.37,64.45 84.79,63.87 84.79,61.79 85.5,61.08 86.62,61.08
N$46
  Top 0.254: R57.2 76.42,168.15 LED_PHASE_2.A
N$47
  Top 0.406: 92.6,61 U$8.1
  Top 0.61: U$6.3 90.98,65.55 92.56,63.97 92.56,61.04 U$8.1
N$48
  Top 0.61: 36.43,41.42 36.43,40.27 37.09,39.61 37.09,38.62 AMC3PWR.3
  Top 0.813: 36.43,41.42 U$11.C C50.1 42.53,41.48 U$17.C
N$49
  Top 0.813: U$11.A 36.48,50.14 U$15.5
N$50
  Top 0.813: U$17.A 42.65,50.15 U$15.8
N$51
  Top 0.61: 36.55,61.05 U$15.4 35.53,61.03 35.23,61.33 35.23,63.77 36.78,65.32 36.81,65.29 38.92,65.29 39.08,65.46 U$12.1
N$52
  Top 0.61: U$15.1 42.52,61.08 42.52,63.77 40.98,65.31 U$12.3
N$96
  Top 0.813: R4.1 R14.2
N$97
  Top 0.813: R15.2 R14.1
N$98
  Top 0.813: R15.1 R32.2
N$99
  Top 0.813: R32.1 R99.2
N$100
  Top 0.813: R99.1 R100.2
N$101
  Top 0.813: R101.2 R100.1
N$102
  Top 0.813: R102.1 R103.2
N$103
  Top 0.813: R104.2 R103.1
N$104
  Top 0.813: R104.1 R105.2
N$105
  Top 0.813: R105.1 R106.2
N$106
  Top 0.813: R106.1 R107.2
N$107
  Top 0.813: R108.2 R107.1
N$108
  Top 0.813: R109.1 R110.2
N$109
  Top 0.813: R111.2 R110.1
N$110
  Top 0.813: R111.1 R112.2
N$111
  Top 0.813: R112.1 R113.2
N$112
  Top 0.813: R113.1 R114.2
N$113
  Top 0.813: R115.2 R114.1
N$114
  Top 0.813: L1.2 R4.2
N$115
  Top 0.813: L3.2 R102.2
N$116
  Top 0.813: L5.2 R109.2
N$117
  Top 0.813: C9.1 R121.1 R123.2 C36.1
N$118
  Top 0.813: C8.1 R118.1 R117.2 C1.1
N$119
  Top 0.813: R125.1 C38.1 | R127.2 C43.1
  Top 1.016: R127.2 R125.1
NEUTRAL
  Top 1.016: L6.1 21.4,82.1 16.5,87 16.5,90.39 R3.1
  Bottom 1.016: 12.96,120.9 12.96,145.11 R1.1 | 12.96,120.9 12.96,119.4 | 12.96,119.4 12.96,117.9 | 12.96,117.9 12.96,99.36 | 12.96,99.36 12.96,97.86 | 12.96,97.86 12.96,96.36 | 12.96,96.36 12.96,93.94 R3.1 | 12.96,99.36 11.46,97.86 | 11.46,97.86 12.96,96.36 | 12.96,97.86 11.46,97.86 | 11.46,97.86 NEUTRAL.TP | 12.96,120.9 14.46,119.4 | 12.96,117.9 14.38,119.32 | 12.96,119.4 14.46,119.4 | 14.46,119.4 14.46,119.5 14.64,119.68 R2.1
PORT_DTR  (via drill 0.5)
  Top 0.406: D7.2 v140.9,154.67
  Bottom 0.406: RS1.4 142.78,154.65 140.92,154.65 v140.9,154.67
PORT_RTS
  Top 0.406: D6.2 143.28,156.25 144.25,157.21 147.76,157.21 149.03,155.94 149.03,155.36 RS1.7
PORT_RX
  Top 0.406: U2.14 142.01,145.22 arc45 142.19,145.3 142.93,146.04 142.93,154.19 arc-45 143,154.37 144.45,155.82 147.06,155.82 arc-45 RS1.2
PORT_TX
  Top 0.406: RS1.3 147.07,153.1 145.29,153.1 144.35,152.16 144.35,145.51 arc-45 144.28,145.33 | U2.13 143.43,144.59 arc45 143.61,144.67 144.05,145.1 144.28,145.33 | 144.28,145.33 144.4,145.45
REACT  (via drill 0.4)
  Top 0.254: LED_REACT.K 97.52,172.38 | 97.52,172.38 97.46,172.38 | 97.07,172.77 60.81,172.77 60.31,172.27 v59.77,172.27 | 97.46,172.38 97.07,172.77 | 97.52,172.38 97.59,172.38 97.98,172.77 99.94,172.77 arc-45 100.12,172.69 106.81,166 106.81,148.76 117.01,138.57 | 98.05,172.77 97.07,172.77 | 97.36,172.61 97.46,172.61 | 97.46,172.61 97.67,172.61 | 97.46,172.38 97.46,172.6 97.46,172.61 | 117.26,138.31 117.01,138.57 | U4.52 109.59,97.12 117.35,104.89 117.35,138.23 117.01,138.57
  Top 0.61: U5.3 38.43,178.47 41.91,181.95 53.32,181.95 REACT.2
  Bottom 0.254: REACT.2 53.52,182.06 55.58,182.06 56.52,181.12 56.52,174 58.25,172.27 v59.77,172.27
RESET
  Top 0.254: 131.5,94.06 R51.2 | 148.34,91.68 JTAG.11
  Top 0.61: 148.34,91.68 146.33,91.68 144.35,89.7 137.57,89.7 JP5.3 136.07,88.2 C53.2 131.49,94.07 R51.2 | 131.44,94.04 R51.2 | R51.2 131.26,93.87 129.19,93.87 124.62,98.44 124.23,98.82 | 124.16,99 arc45 124.23,98.82 | RESET.1 123.14,99.91 124.23,98.82
RS232_RXD  (via drill 0.2)
  Top 0.254: U4.16 88.4,101.14 v89.06,101.79
  Bottom 0.254: v89.06,101.79 89.06,105.98 arc-45 89.13,106.16 90.58,107.61 92.71,107.61 arc-45 92.89,107.53 97.72,102.71 110.69,102.71 arc45 110.87,102.78 113.62,105.53 arc-45 113.64,105.57 114.58,106.52 114.79,106.72 | 114.79,106.72 114.86,106.8 | JP15.1 arc45 146.54,117.67 146.54,116.3 145.47,115.23 arc-45 145.29,115.15 142.55,115.15 134.27,106.87 arc-45 134.09,106.8 114.97,106.8 arc45 114.79,106.72
RS232_TXD  (via drill 0.2)
  Top 0.254: U4.17 89.18,100.63 arc45 v89.28,100.67
  Bottom 0.254: v89.28,100.67 arc45 89.33,100.69 90.02,101.39 90.02,106 arc-45 90.1,106.18 90.96,107.05 92.48,107.05 arc-45 92.53,107.03 97.39,102.17 111.23,102.17 arc45 111.41,102.25 114.51,105.35 136.68,105.35 arc45 136.86,105.42 142.68,111.24 arc-45 142.86,111.32 150.09,111.32 152.76,113.98 arc45 152.84,114.17 JP16.1
RXD_IN
  Top 0.406: U1.2 arc45 139.63,130.61 139.63,124.22 arc45 139.7,124.04 144.05,119.7 JP15.2
S0
  Top 0.254: LCD1.1 51.33,134.23 60.48,125.07 88.75,125.07 91.66,122.17 U4.94
S1
  Top 0.254: LCD1.2 53.84,134.23 62.5,125.57 89,125.57 92.17,122.41 U4.93
S2
  Top 0.254: LCD1.3 56.34,134.23 64.5,126.07 89.25,126.07 92.65,122.67 U4.92
S3
  Top 0.254: LCD1.4 66.5,126.57 89.5,126.57 93.16,122.92 U4.91
S4
  Top 0.254: LCD1.5 61.38,134.19 68.5,127.07 89.75,127.07 93.67,123.16 U4.90
S5
  Top 0.254: LCD1.6 63.92,134.15 70.5,127.57 90,127.57 94.15,123.43 U4.89
S6
  Top 0.254: LCD1.7 66.46,134.11 72.5,128.07 90.25,128.07 94.66,123.67 U4.88
S7
  Top 0.254: LCD1.8 69,134.07 74.5,128.57 90.5,128.57 95.16,123.91 U4.87
S8
  Top 0.254: LCD1.9 71.54,134.03 76.5,129.07 90.75,129.07 95.65,124.18 U4.86
S9
  Top 0.254: LCD1.10 74.08,133.99 78.5,129.57 91,129.57 96.15,124.42 U4.85
S10
  Top 0.254: LCD1.11 76.62,133.95 80.5,130.07 91.25,130.07 96.66,124.66 U4.84
S11
  Top 0.254: LCD1.12 79.16,133.91 82.5,130.57 91.5,130.57 97.14,124.93 U4.83
S12
  Top 0.254: LCD1.13 81.7,133.9 84.5,131.07 91.75,131.07 97.65,125.17 U4.82
S13
  Top 0.254: LCD1.14 84.24,133.83 86.5,131.57 92,131.57 98.16,125.41 U4.81
S14
  Top 0.254: LCD1.15 86.78,133.82 88.5,132.07 92.25,132.07 98.64,125.68 U4.80
S15
  Top 0.254: LCD1.16 89.32,133.78 90.5,132.57 92.5,132.57 99.15,125.92 U4.79
S16
  Top 0.254: LCD1.17 91.86,133.99 99.38,126.45 99.66,126.17 U4.78
S17
  Top 0.254: LCD1.18 94.4,132.13 99.88,126.7 100.17,126.4 U4.77
S18
  Top 0.254: LCD1.19 96.94,130.41 100.38,126.95 100.65,126.68 U4.76
S19
  Top 0.254: U4.73 104.39,107.64 106.75,110 106.75,127.21 LCD1.20
S20
  Top 0.254: LCD1.21 102.09,134.23 107.25,129.07 107.25,109.75 104.63,107.13 U4.72
S21
  Top 0.254: LCD1.22 104.61,134.27 106.56,134.27 106.75,134.08 106.75,134.07 107.76,133.06 107.76,109.51 104.87,106.62 U4.71
S22  (via drill 0.2, 0.36)
  Top 0.254: v103.25,138.07 103.75,138.07 108.25,133.58 108.25,109.25 105.14,106.14 U4.70 | v103.25,152.57 103.25,162.89 LCD1.23
  Bottom 0.254: v103.25,138.07 v103.25,152.57
S23  (via drill 0.2, 0.36)
  Top 0.254: v102.25,139.07 103.5,139.07 108.75,133.82 108.75,109 105.38,105.63 U4.69 | v102.25,153.57 102.25,163.97 LCD1.24
  Bottom 0.254: v102.25,139.07 v102.25,153.57
S24  (via drill 0.36)
  Top 0.254: v101.25,140.07 103.25,140.07 109.26,134.06 109.26,108.77 105.59,105.12 U4.68
  Bottom 0.254: v101.25,140.07 101.25,152.07 89.32,163.96 LCD1.29
S25  (via drill 0.36)
  Top 0.254: v100.25,141.07 103,141.07 109.74,134.33 109.74,108.5 105.88,104.64 U4.67
  Bottom 0.254: v100.25,141.07 100.25,152.32 90,162.57 88.25,162.57 86.78,164.04 LCD1.30
S26  (via drill 0.36)
  Top 0.254: v99.25,142.07 102.75,142.07 110.25,134.57 110.25,108.26 106.13,104.13 U4.66
  Bottom 0.254: v99.25,142.07 99.25,152.57 89.75,162.07 86.25,162.07 84.24,164.08 LCD1.31
S27  (via drill 0.36)
  Top 0.254: v98.25,143.07 102.5,143.07 110.76,134.81 110.76,108.02 106.37,103.63 U4.65
  Bottom 0.254: v98.25,143.07 98.25,152.82 89.5,161.57 84.25,161.57 81.7,164.12 LCD1.32
S28  (via drill 0.36)
  Top 0.254: v97.25,144.07 102.25,144.07 111.24,135.08 111.24,107.75 106.64,103.14 U4.64
  Bottom 0.254: v97.25,144.07 97.25,153.07 89.25,161.07 82.25,161.07 79.16,164.16 LCD1.33
S29  (via drill 0.36)
  Top 0.254: v96.25,145.07 102,145.07 111.75,135.32 111.75,107.51 106.87,102.64 U4.63
  Bottom 0.254: v96.25,145.07 96.25,153.32 89,160.57 80.25,160.57 LCD1.34
S30  (via drill 0.36)
  Top 0.254: v95.25,146.07 101.75,146.07 112.26,135.57 112.26,107.27 107.11,102.13 U4.62
  Bottom 0.254: v95.25,146.07 95.25,153.57 88.75,160.07 78.25,160.07 74.12,164.2 LCD1.35
S31  (via drill 0.36)
  Top 0.254: v94.25,147.07 101.5,147.07 112.74,135.83 112.74,107.01 107.38,101.64 U4.61
  Bottom 0.254: v94.25,147.07 94.25,153.82 88.5,159.57 76.25,159.57 71.62,164.2 LCD1.36
S32  (via drill 0.36)
  Top 0.254: v93.25,148.07 101.25,148.07 113.25,136.07 113.25,106.77 107.61,101.14 U4.60
  Bottom 0.254: v93.25,148.07 93.25,154.07 88.25,159.07 74.25,159.07 69.12,164.2 LCD1.37
S33  (via drill 0.36)
  Top 0.254: v92.25,149.07 101,149.07 113.76,136.32 113.76,106.53 107.85,100.63 U4.59
  Bottom 0.254: v92.25,149.07 92.25,154.32 88,158.57 72.25,158.57 66.62,164.2 LCD1.38
S34  (via drill 0.36)
  Top 0.254: v91.25,150.07 100.75,150.07 114.24,136.58 114.24,106.27 108.12,100.15 U4.58
  Bottom 0.254: v91.25,150.07 91.25,154.57 87.75,158.07 70,158.07 63.92,164.15 LCD1.39
S35  (via drill 0.36)
  Top 0.254: v90.25,151.07 100.5,151.07 114.75,136.83 114.75,106.03 108.36,99.64 U4.57
  Bottom 0.254: v90.25,151.07 90.25,154.82 87.5,157.57 68,157.57 LCD1.40
S36  (via drill 0.36)
  Top 0.254: U4.56 108.6,99.13 115.25,105.78 115.25,137.07 100.25,152.07 v89.25,152.07
  Bottom 0.254: LCD1.41 59.12,164.2 66.25,157.07 87,157.07 89.25,154.82 v89.25,152.07
S37  (via drill 0.36)
  Top 0.254: U4.55 108.87,98.65 115.75,105.53 115.75,137.32 100,153.07 v88.25,153.07
  Bottom 0.254: LCD1.42 56.62,164.2 64.25,156.57 86.75,156.57 88.25,155.07 v88.25,153.07
S38  (via drill 0.36)
  Top 0.254: U4.54 109.11,98.14 116.25,105.28 116.25,137.57 99.75,154.07 v87.25,154.07
  Bottom 0.254: LCD1.43 53.87,164.2 62.03,156.05 86.44,156.05 87.25,155.24 v87.25,154.07
S39  (via drill 0.4)
  Top 0.254: U4.53 109.33,97.63 116.84,105.14 116.84,107.43 116.84,137.94 116.69,138.09 116.6,138.18 99.72,155.06 v85.88,155.06
  Bottom 0.254: v85.88,155.06 59.95,155.06 51.22,163.78 LCD1.44
TCK
  Top 0.61: JTAG.7 143.97,92.39 137.62,92.39 JP6.3 136.16,91.06 R48.1
TDI
  Top 0.254: 148.26,101.77 JTAG.3
  Top 0.61: JP8.3 136.25,96.94 137.01,97.7 142.01,97.75 145.98,101.77 148.26,101.77
TDO  (via drill 0.4)
  Top 0.254: 148.26,104.31 JTAG.1 148.24,104.28
  Top 0.61: 148.24,104.28 134.47,104.28 arc45 134.3,104.21 132.72,102.63 v132.72,100.14
  Bottom 0.61: JP5.1 142.5,89.55 142.5,99.78 142.08,100.2 arc45 141.9,100.28 138.08,100.28 136.87,99.07 arc-45 136.69,99 JP9.3 arc45 136.13,99.05 133.48,99.05 132.79,99.74 arc-45 132.72,99.92 v132.72,100.14
TEST/SBWTCK  (via drill 0.2, 0.4)
  Top 0.254: U4.95 91.15,107.55 v92.79,105.91
  Top 0.61: v142.96,103.14 149.15,103.14 149.21,103.08 arc45 149.25,103.06 149.54,102.78 arc-45 149.61,102.6 149.61,98.11 150.89,96.83 arc-45 JTAG.8
  Bottom 0.254: v92.79,105.91 96.93,101.77 96.93,101.74 96.98,101.69 111.92,101.69 115.07,104.84 129.57,104.84 133.1,104.84 JP4.3
  Bottom 0.61: JP4.3 JP4.2 140.16,103.06 arc-45 140.34,103.14 v142.96,103.14
TMS
  Top 0.254: 148.29,99.4 JTAG.5
  Top 0.61: JP7.3 136.22,94.3 136.99,95.06 141.94,95.06 146.28,99.4 148.29,99.4
TXD_IN
  Top 0.406: U1.3 140.92,124.76 arc45 141,124.58 145.75,119.83 148.16,119.83 arc-45 148.34,119.75 JP16.2
V1_IN
  Top 0.254: U4.11 87.03,103.62 76.97,103.62 76.13,104.46
  Top 0.813: R116.2 56.73,123.85 76.13,104.46
V2_IN
  Top 0.254: U4.12 | 87.01,103.12 U4.12 | U4.12 86.23,103.14 86.21,103.16 74.6,103.16 74.19,103.58 73.94,103.82
  Top 0.813: R120.2 63.41,114.35 74.19,103.58
V3_IN
  Top 0.254: U4.13 72.36,102.64 72.11,102.88 | 53.17,104.85 53.23,104.92 53.26,104.85
  Top 0.813: R124.2 53.17,104.85 | 53.26,104.85 70.06,104.85 72.11,102.88
VASYS
  Top 0.254: U4.10 81.89,104.13 80.94,105.08 C28.1 C32.1
VCC_RS232
  Top 0.254: U1.8 138.38,136.94 138,137.33 C64.1 136.83,137.34 136.83,138.34 135.55,139.62 130.3,139.62
  Top 0.406: U2.16 138.89,147.63 C61.1 | 138.87,147.65 C61.1 | C56.1 arc-45 131.25,151.67 U3.5 130.21,152.84 arc-45 130.03,152.92 129.57,153.38 129.57,161.31 arc45 JP14.1 | C56.1 137.06,151.57 arc-45 137.24,151.5 138.81,149.92 138.81,147.79 arc45 C61.1 | U1.8 138.33,135.67 arc45 138.26,135.85 | C56.1 arc-45 131.35,151.42 131.35,150.33 130.35,149.34 arc-45 130.18,149.26 129.01,149.26 128.32,148.58 arc45 128.25,148.4 128.25,141.57 130.12,139.7 arc45 130.3,139.62
VCORE
  Top 0.254: U4.23 87.03,97.63 85.42,97.63 84.99,97.19 84.99,94.78 83.27,93.05 82.31,93.05 C33.1
VDSYS  (via drill 0.2)
  Top 0.254: 80.95,95.21 C15.1 | v89.97,96.53 89.97,98.72 | 89.97,98.72 89.94,98.74 | 90.35,99.15 92.71,99.15 94,100.49 94,108 94.75,108.75 99.17,108.75 99.83,108.15 U4.74 103.77,108.15 104.63,109 104.63,110.17 C18.1 | 89.97,98.72 89.97,98.77 | 89.97,98.77 90.35,99.15 | 89.97,98.77 89.92,98.77 89.54,99.15 | 89.54,99.15 90.35,99.15 | 89.77,99 90.02,99 | 90.02,99 90.07,99 | 89.97,98.77 89.97,98.95 90.02,99 | R7.1 92.95,91.16 v92.94,91.17 | 87.03,99.12 U4.20 | 89.54,99.15 87.06,99.15 U4.20 | U4.20 84.29,99.13 83.9,98.74 83.9,96.13 82.91,95.14 80.93,95.14 C15.1 | C14.1 C15.1
  Bottom 0.254: 89.94,96.51 v89.97,96.53 90,96.51 90,95.03 92.57,92.46 92.94,92.09 v92.94,91.17
VREF
  Top 0.254: C30.1 85.89,105.63 U4.7
XIN
  Top 0.254: XT1.P2 84.38,91.54 84.38,93.31 85.47,94.4 85.47,96.58 86.02,97.12 U4.24 | 84.42,91.5 XT1.P2 | C37.1 82.79,90.65 83.39,91.25 84.34,91.25 XT1.P2
XOUT
  Top 0.254: C40.1 88.37,90.97 87.93,91.41 XT1.P1 86.92,91.5 86.92,93.38 85.96,94.35 85.96,96.36 86.24,96.64 U4.25

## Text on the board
tPlace: + 3.3V - | 1 | + | + | + | + | + | RS232_3.3 | RS232_GND | 50/60 Hz | High Voltage | Danger | 120/240 Vrms | 50/60 Hz | 120/240 Vrms | High Voltage | Danger | 50/60 Hz | 120/240 Vrms | AMC_CLK | BITSTREAM_I3 | AMC_CLK | BITSTREAM_I1 | AMC_CLK | BITSTREAM_I2 | L | A | L | A | L | A | Danger | Danger | I | I | I | High Voltage | High Voltage | E | E | E | 50 mV MAX | 50 mV MAX | 50 mV MAX | + V - | + V - | + V -
tNames: DGND | DGND | ISOLATED | REACT | ACT | ISO_GND | ISO_REA | ISO_ACT | ACTIVE | PHASE 1 | PHASE 2 | PHASE 3 | REACTIVE | ISO_VCC | + | DVCC | EXTERNAL | RX-EN | TX-EN | INTERNAL | RS-232 | SBW | JTAG | 1 | TIDM-ISO-SHUNT-EMTR | Version 1.0 | M. MESGANAW / JAN 2015 | For more designs, visit www.ti.com/smartgrid
_tplace: DGND | DGND | C67 | ISOLATED | REACT | ACT | DVCC | DGND | C66 | ISO_GND | + 3.3V - | ISO_REA | * | ISO_ACT | U5 | ACTIVE | PHASE 1 | PHASE 2 | PHASE 3 | REACTIVE | ISO_VCC | ISO_PULSE | + | + | + | + | + | R58 | R22 | R57 | R21 | R20 | RS1 | RS232_3.3 | RS232_GND | C54 | 1 | L1 | R15 | R32 | R101 | D6 | 6 | U3 | C55 | 2 | 7 | D7 | * | 3 | 8 | C56 | LINE_1 | 50/60 Hz | 4 | R4 | R14 | R99 | R100 | High Voltage | C60 | C61 | 9 | 5 | LCD1 | * | Danger | C62 | R1 | C57 | C63 | U2 | 120/240 Vrms | C64 | LINE_2 | U1 | L3 | R104 | R105 | R108 | * | R36 | C65 | 50/60 Hz | 120/240 Vrms | R116 | D45 | R119 | R102 | R103 | R106 | R107 | High Voltage | R118 | C8 | D44 | DVCC | R117 | C1 | LINE_3 | EXTERNAL | R2 | Danger | R120 | RX-EN | TX-EN | D47 | C31 | C29 | INTERNAL | RS-232 | R122 | C30 | C18 | 50/60 Hz | D46 | R121 | C9 | C32 | C28 | 120/240 Vrms | R123 | C36 | 1 | 2 | R124 | SBW | D49 | JTAG | R126 | C7 | C6 | R5 | C4 | C5 | NEUTRAL | R6 | U4 | RESET | L5 | R111 | R115 | R125 | C38 | R112 | D48 | R127 | C43 | 14 | C16 | C17 | C14 | C15 | R49 | R51 | C58 | C49 | TIDM-ISO-SHUNT-EMTR | C33 | R109 | R110 | R113 | R114 | C59 | R48 | C53 | R7 | R3 | C37 | C40 | BTN1 | JTAG | XT1 | L6 | AMC_CLK | BITSTREAM_I3 | AMC_CLK | BITSTREAM_I1 | U$12 | AMC_CLK | BITSTREAM_I2 | U$6 | U$10 | JP3 | C22 | C47 | JP1 | C42 | C52 | R16 | JP2 | C27 | 1 | C25 | 1 | C23 | 1 | C34 | C41 | CLOCK_GENERATOR | C26 | C46 | C24 | C51 | 1 | 1 | 1 | U$15 | XFR | XFR | U$8 | XFR | U$16 | AMC | U$4 | AMC | U$3 | AMC | U$2 | 1 | 1 | 1 | C21 | C19 | C12 | L | A | L | A | CSEL2 | L | A | CSEL1 | CSEL3 | C10 | C20 | C3 | C13 | C2 | C11 | U$11 | C50 | U$17 | Danger | U$5 | C45 | U$9 | Danger | U$1 | C39 | U$19 | R140 | R138 | R136 | R139 | AMC3PWR | I | R137 | AMC2PWR | I | R135 | AMC1PWR | I | High Voltage | High Voltage | R/L3 | TVS3 | R/L4 | R/L1 | TVS1 | R/L2 | R/L9 | TVS2 | R/L10 | E | E | E | C48 | C44 | C35 | D14 | U$14 | D2 | U$7 | D11 | U$13 | D35 | D10 | D12 | D13 | D15 | D1 | D5 | D3 | D4 | Version 1.0 | M. MESGANAW / JAN 2015 | For more designs, visit www.ti.com/smartgrid | I3+ | I3- | I3LIVE | I2+ | I2- | I2LIVE | I1+ | I1- | I1LIVE | 50 mV MAX | 50 mV MAX | 50 mV MAX | 1 | 2 | 1 | 2 | 1 | 2 | + V - | + V - | + V -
